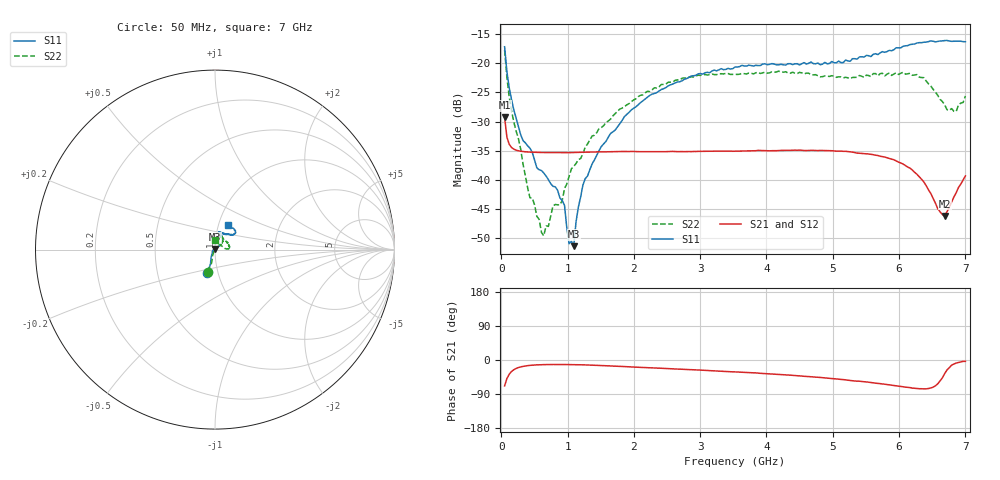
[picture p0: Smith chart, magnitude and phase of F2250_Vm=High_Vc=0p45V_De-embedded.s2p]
! Integrated Device Technology
! Corporate Headquarters
! 6024 Silver Creek Valley Road
! San Jose, CA 95138  USA
! Phone:  1-408-284-8200
! Toll Free:  1-800-223-1366
! Webpage:  http://www.idt.com/
! Timing and RF Division
! 515 Groton Road, Suite 102
! Westford, MA 01886-6024
! Device:  F2250
! Description: Voltage Variable RF Attenuator
! Frequency:  50.0 -  6000.00 MHz
! Package:  3x3 mm Thin QFN Plastic Package: 16 pin
! Ports:  2 RF, 3 DC
!  Pin  1  = GND
!  Pin  2  = NC
!  Pin  3  = RF1  = Port 1
!  Pin  4  = NC
!  Pin  5  = GND
!  Pin  6  = GND
!  Pin  7  = GND
!  Pin  8  = GND
!  Pin  9  = NC
!  Pin 10  = RF2  = Port 2
!  Pin 11  = NC
!  Pin 12  = GND
!  Pin 13  = GND
!  Pin 14  = VCNTRL
!  Pin 15  = VDD
!  Pin 16  = VMODE
! Vcntrl:  0.450 Volts
! Vmode:  +3.300 Volts
! Vdd:  +3.30  Volts
! Current:  1.264 mA
! Data:  The device was measured on a the F2250 evaluation board which has
!  individual transmission lines to the RF pins.  Data was collected
!  using a calibrated network analyzer.  The evaluation board was
!  de-embedded using a TRL calibration technique.
!  The reference plane is the edge of the package pin.
! Misc:  SN 10
!  Action Tracker AT0258
! Date Measured:  2014-11-26
! Date:  2015-10-15  MJV
! Note:
!  Integrated Device Technology supplies this data as a sample of measured
!  data at the package pin for this product.  Your particular data for this
!  product may vary.
!  Data was taken at 25 degrees C.
!  Integrated Device Technology reserves the right to change this data at anytime.
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# GHz S dB R 50
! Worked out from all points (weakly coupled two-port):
!   201 points, 50 MHz to 7 GHz, reference 50 ohm
!   highest |S21| = -29.28 dB at 50 MHz (marker M1); lowest = -46.1 dB at 6.687 GHz (marker M2)
!   lowest |S11| = -51.3 dB at 1.093 GHz (marker M3), VSWR 1.01, Z = 50 + j0.272 ohm
!   |S11| at or under -10 dB: start of sweep to end of sweep
!   |S22| runs from -49.5 to -17.8 dB; largest |S21 - S12| = 5.7e-05
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0.05  -17.17 -108.5  -29.28 -68.3  -29.28 -68.3  -17.77 -108.6
0.1195  -24.20 -111.9  -33.88 -37.5  -33.87 -37.5  -25.76 -107.0
0.29325  -32.26 -127.3  -35.07 -18.1  -35.07 -18.1  -34.75 -114.1
0.43225  -34.55 -145.2  -35.21 -14.2  -35.21 -14.2  -43.02 -147.7
0.606  -38.37 -162.4  -35.28 -12.4  -35.28 -12.4  -48.97 165.8
0.71025  -39.92 -167.5  -35.30 -12.0  -35.30 -12.0  -47.93 114.9
0.77975  -41.07 176.3  -35.31 -11.9  -35.30 -11.9  -44.42 101.3
0.91875  -43.50 156.0  -35.31 -11.9  -35.31 -11.9  -43.53 76.4
0.9535  -44.32 170.4  -35.31 -12.0  -35.31 -11.9  -41.45 83.2
1.023  -50.90 140.3  -35.30 -12.0  -35.30 -12.1  -39.34 67.7
1.0925  -51.32 89.4  -35.29 -12.2  -35.29 -12.2  -37.68 62.9
1.12725  -47.18 60.9  -35.28 -12.4  -35.27 -12.3  -37.18 56.7
1.2315  -40.84 40.6  -35.24 -12.7  -35.24 -12.7  -35.48 47.3
1.6485  -32.02 41.1  -35.16 -15.5  -35.16 -15.5  -29.56 45.3
2.37825  -24.75 46.6  -35.13 -21.5  -35.13 -21.6  -24.07 46.2
3.525  -20.65 71.7  -35.06 -31.4  -35.06 -31.4  -21.87 68.9
4.7065  -20.06 72.0  -34.92 -44.8  -34.91 -44.8  -21.99 68.0
5.85325  -17.79 40.5  -36.31 -65.6  -36.31 -65.7  -21.67 19.4
6.3745  -16.40 40.9  -40.35 -76.3  -40.35 -76.3  -22.47 3.2
6.68725  -16.12 47.8  -46.13 -36.0  -46.12 -35.7  -27.10 25.1
6.861  -16.22 54.5  -42.17 -8.1  -42.12 -8.1  -28.26 58.3
7  -16.32 62.4  -39.29 -3.5  -39.26 -3.7  -25.62 87.0
